TYPE LstPressure :
STRUCT
    ToleranceMode:STRING;		//'Value' or 'Percent'
	ToleranceDelayTime:INT;
	PressureUnitMode:STRING;	//'Pressure' or 'Position'
	StartValue:INT;
	StartValueWarningRange:INT;
	StartValueAlarmRange:INT;
	ValvePositionPreset:INT;
	EnableRamp:BOOL;
	HoldTime:INT;
	RampTime:INT;
	TargetValue:INT;
END_STRUCT
END_TYPE
